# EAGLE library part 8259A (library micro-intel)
MICROCOMPUTER/PERIPHERAL DEVICE
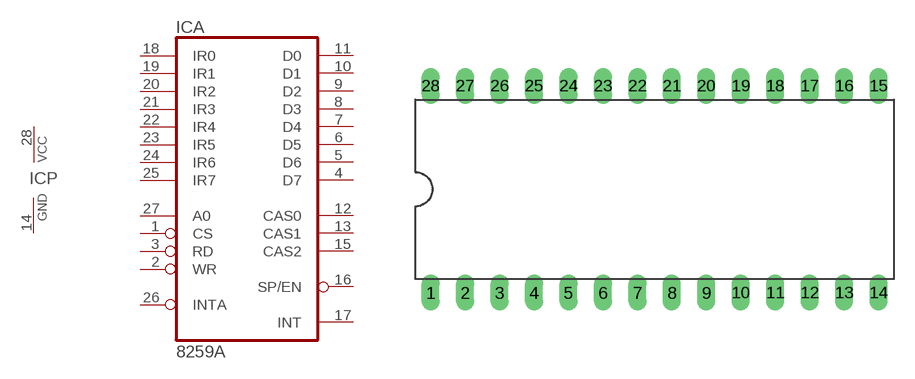
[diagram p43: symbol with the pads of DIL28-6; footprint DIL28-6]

Designator prefix IC; gates A=8259A P=PWRN

## 8259A (OC_FARNELL: unknown; OC_NEWARK: unknown)  [DIL28-6]
1  A:CS  in
2  A:WR  in
3  A:RD  in
4  A:D7
5  A:D6
6  A:D5
7  A:D4
8  A:D3
9  A:D2
10  A:D1
11  A:D0
12  A:CAS0
13  A:CAS1
14  P:GND  pwr
15  A:CAS2
16  A:SP/EN
17  A:INT  out
18  A:IR0  in
19  A:IR1  in
20  A:IR2  in
21  A:IR3  in
22  A:IR4  in
23  A:IR5  in
24  A:IR6  in
25  A:IR7  in
26  A:INTA  in
27  A:A0  in
28  P:VCC  pwr

## Footprint DIL28-6 (pad centres in mm)
Dual In Line Package 0.6 inch
drill 0.813 long: 1 -16.51,-7.62; 2 -13.97,-7.62; 3 -11.43,-7.62; 4 -8.89,-7.62; 5 -6.35,-7.62; 6 -3.81,-7.62; 7 -1.27,-7.62; 8 1.27,-7.62; 9 3.81,-7.62; 10 6.35,-7.62; 11 8.89,-7.62; 12 11.43,-7.62; 13 13.97,-7.62; 14 16.51,-7.62; 15 16.51,7.62; 16 13.97,7.62; 17 11.43,7.62; 18 8.89,7.62; 19 6.35,7.62; 20 3.81,7.62; 21 1.27,7.62; 22 -1.27,7.62; 23 -3.81,7.62; 24 -6.35,7.62; 25 -8.89,7.62; 26 -11.43,7.62; 27 -13.97,7.62; 28 -16.51,7.62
